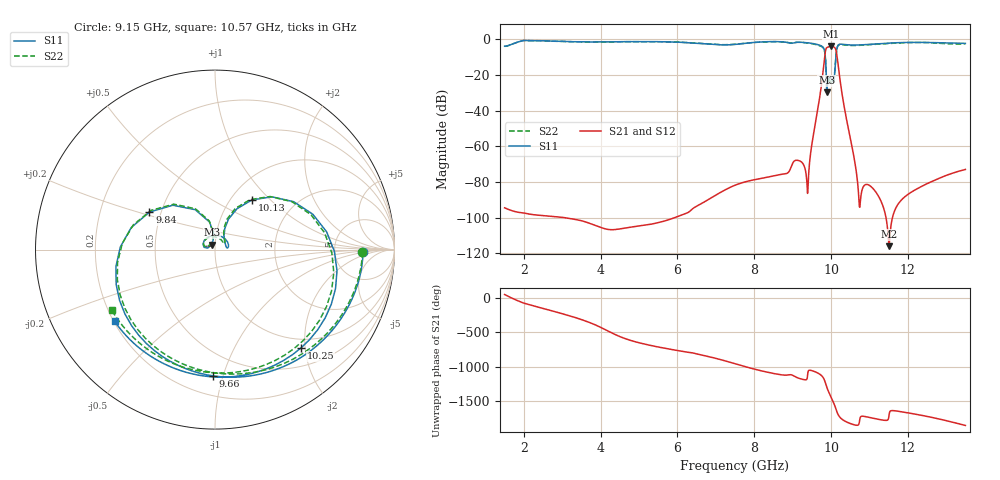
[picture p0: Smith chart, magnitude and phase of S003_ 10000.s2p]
# Hz S DB R 50
! Planar, S50180, , 20.4.1/1
! Date: 14.12.2021 19:04:02
! Data: Format (Calibration Info)
! Freq	S11:dB/Ang(--)	S21:dB/Ang(--)	S12:dB/Ang(--)	S22:dB/Ang(--)
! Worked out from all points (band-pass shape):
!   1201 points, 1.5 GHz to 13.5 GHz, reference 50 ohm
!   highest |S21| = -4.06 dB at 10 GHz (marker M1); lowest = -115.9 dB at 11.51 GHz (marker M2)
!   |S21| within 3 dB of the highest: 9.853 GHz to 10.14 GHz (285.1 MHz wide, 2.85 % of centre)
!   lowest |S11| = -29.7 dB at 9.89 GHz (marker M3), VSWR 1.07, Z = 48.3 + j2.69 ohm
!   |S11| at or under -10 dB: 9.852 GHz to 10.13 GHz (274.7 MHz wide, 2.75 % of centre)
!   |S22| runs from -27.6 to -0.7 dB; largest |S21 - S12| = 2.2e-06
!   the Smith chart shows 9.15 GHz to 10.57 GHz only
!   S11 on the Smith chart (normalised r, x): 9.15 GHz: 10, -1; 9.66 GHz: 0.33, -0.93; 9.84 GHz: 0.43, +0.22; 10.13 GHz: 1.24, +0.78; 10.25 GHz: 0.83, -1.92; 10.57 GHz: 0.20, -0.31
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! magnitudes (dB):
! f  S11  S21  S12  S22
! 1.5 GHz  -3.9  -94.4  -94.4  -4.0
! 3.5 GHz  -1.4  -101.7  -101.7  -1.4
! 5.5 GHz  -1.4  -102.8  -102.8  -1.4
! 7.5 GHz  -2.9  -81.8  -81.8  -2.8
! 8.82 GHz  -1.7  -75.4  -75.4  -1.7
! 9.15 GHz  -1.7  -67.9  -67.9  -1.7
! 9.38 GHz  -2.0  -83.1  -83.1  -2.1
! 9.5 GHz  -2.3  -59.1  -59.1  -2.5
! 9.66 GHz  -3.1  -38.7  -38.7  -3.3
! 9.79 GHz  -4.4  -18.7  -18.7  -4.6
! 9.84 GHz  -7.5  -9.0  -9.0  -7.6
! 9.89 GHz  -29.7  -4.7  -4.7  -27.6
! 10 GHz  -21.9  -4.1  -4.1  -24.5
! 10.06 GHz  -23.9  -4.2  -4.2  -23.0
! 10.13 GHz  -9.3  -6.3  -6.3  -9.4
! 10.25 GHz  -2.8  -25.1  -25.1  -3.0
! 10.57 GHz  -3.3  -62.8  -62.8  -3.5
! 10.74 GHz  -3.2  -93.9  -93.9  -3.4
! 11.5 GHz  -2.2  -113.7  -113.7  -2.4
! 11.51 GHz  -2.1  -115.9  -115.9  -2.4
! 12.58 GHz  -1.8  -80.2  -80.2  -2.0
! 13.5 GHz  -2.3  -73.0  -73.0  -2.6
